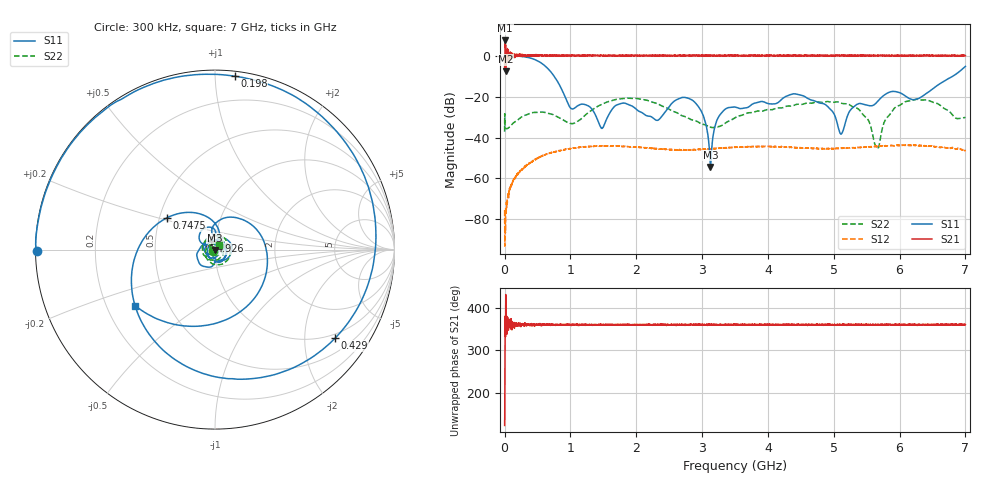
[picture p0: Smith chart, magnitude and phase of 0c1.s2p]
!Keysight Technologies,N5232A,MY52221221,A.10.65.11
!Date: Wednesday, October 16, 2024 11:59:15
!Correction: S11(Full 2 Port(1,4))
!S41(Full 2 Port(1,4))
!S14(Full 2 Port(1,4))
!S44(Full 2 Port(1,4))
!S2P File: Measurements: S11, S41, S14, S44:
# Hz S  RI  R 50
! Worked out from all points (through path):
!   4001 points, 300 kHz to 7 GHz, reference 50 ohm
!   highest |S21| = 7.36 dB at 10.8 MHz (marker M1); lowest = -7.8 dB at 16.05 MHz (marker M2)
!   lowest |S11| = -54.3 dB at 3.127 GHz (marker M3), VSWR 1.00, Z = 50 - j0.192 ohm
!   |S11| at or under -10 dB: 750.6 MHz to 6.813 GHz (6.062 GHz wide, 160 % of centre)
!   |S22| runs from -45.3 to -20.8 dB; largest |S21 - S12| = 2.3
!   S11 on the Smith chart (normalised r, x): 300 kHz: 0.00, -0.01; 198 MHz: 0.03, +1.12; 429 MHz: 0.88, -2.80; 747.5 MHz: 0.55, +0.22; 4.926 GHz: 0.95, +0.09; 7 GHz: 0.32, -0.29
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300000  -0.9944 -0.0105  -0.2588 0.39  3.21e-05 0.000166  -0.0115 -0.00778
1.079955e7  -0.9951 0.0913  2.232 0.6828  6.22e-05 0.000127  -0.0166 0.00221
1.604932e7  -0.9888 0.1367  0.3178 0.2579  -4.83e-06 0.000185  -0.0163 0.00333
1.980415e8  0.1094 0.9664  0.9686 0.0219  0.000668 0.00112  0.00281 0.0266
4.290316e8  0.6696 -0.4925  0.9814 -0.0244  0.00247 0.00109  0.037 0.0167
6.022742e8  -0.3999 -0.4193  1.016 0.00539  0.00368 -0.000192  0.0398 -0.0108
7.47518e8  -0.2685 0.1765  1.001 0.00695  0.00392 -0.00198  0.0219 -0.0279
1.1675e9  0.0304 0.0576  1 -0.00156  7.66e-05 -0.00578  -0.0196 0.0213
1.475487e9  0.0166 0.000799  1.003 -0.00596  -0.00426 -0.00454  0.0461 0.0448
1.790473e9  0.0495 -0.0478  1.011 0.00529  -0.00606 -0.000429  0.0822 -0.0339
2.3347e9  0.00117 0.0267  0.998 -0.00598  -0.00259 0.00461  -0.0486 -0.0439
2.838678e9  0.0673 -0.0507  0.9886 0.0179  0.00172 0.00469  0.0105 0.025
3.127416e9  5.58e-05 -0.00192  0.9843 0.00142  0.00387 0.00354  0.0123 -0.013
3.251661e9  0.0179 -0.0264  1.01 -0.00584  0.00473 0.00274  -0.0053 -0.0176
3.50015e9  -0.055 0.00761  0.9829 -0.00143  0.00582 6.97e-05  -0.0276 0.012
4.66735e9  -0.0805 0.0129  1.011 -0.00737  -0.00386 -0.00382  -0.0687 -0.0049
4.926339e9  -0.0224 0.0482  0.9999 0.00159  -0.00508 -0.00177  -0.0385 0.0642
5.113581e9  0.011 -0.00554  1.014 -0.000937  -0.00547 -6.11e-05  0.0138 0.0677
5.656058e9  -0.066 0.0304  0.9973 0.00651  -0.00301 0.00515  -0.00179 -0.00551
5.83455e9  -0.0828 0.0945  0.9997 0.022  -0.000964 0.00621  -0.0247 0.0231
6.795259e9  0.2912 -0.0877  1.001 0.00656  0.00461 -0.00308  0.0358 0.0094
7e9  -0.4442 -0.3117  0.9977 0.00695  0.0014 -0.00463  0.0209 0.0229
